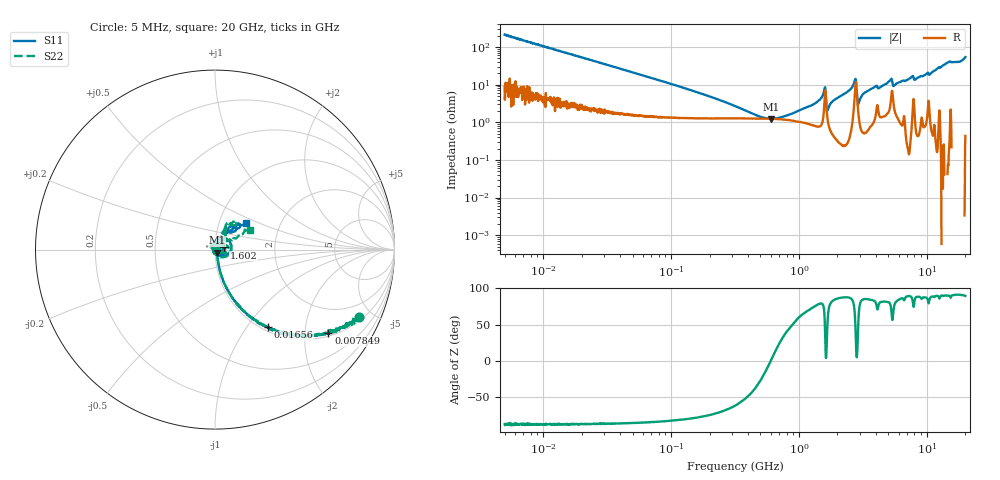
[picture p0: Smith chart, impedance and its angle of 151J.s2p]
!Keysight Technologies,P5008B,MY61100088,A.16.20.02
!Date: Wednesday, November 08, 2023 15:34:21
!Correction: S11(C  2-Port  )
!S21(C  2-Port  )
!S12(C  2-Port  )
!S22(C  2-Port  )
!S2P File: Measurements: S11, S21, S12, S22:Log Frequency Sweep
# Hz S  dB  R 50
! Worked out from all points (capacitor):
!   1601 points, 5 MHz to 20 GHz, reference 50 ohm
!   read as one part in series: C = 153 pF near 5.212 MHz
!   lowest |Z| = 1.23 ohm at 604.5 MHz (marker M1)
!   series resonance near 602.5 MHz, so ESL is about 460 pH
!   S11 on the Smith chart (normalised r, x): 5 MHz: 1.17, -4.19; 7.849 MHz: 1.09, -2.64; 16.56 MHz: 1.06, -1.27; 1.602 GHz: 1.11, +0.03; 20 GHz: 1.35, +0.42
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5000000  -1.03 -25.1  -7.45 62.5  -7.45 62.6  -1.03 -25.0
7849320  -2.11 -36.4  -4.54 51.6  -4.54 51.6  -2.11 -36.4
1.655836e7  -5.60 -55.5  -1.67 31.6  -1.66 31.6  -5.60 -55.6
1.995555e7  -6.76 -60.2  -1.23 27.3  -1.22 27.3  -6.76 -60.2
7.964482e7  -17.66 -76.7  -0.19 7.3  -0.19 7.3  -17.79 -77.0
3.162278e8  -29.20 -67.3  -0.12 1.1  -0.12 1.1  -31.44 -64.0
6.045204e8  -33.94 -58.0  -0.12 -0.6  -0.12 -0.6  -39.88 -13.4
1.2621e9  -44.82 -86.5  -0.14 -2.8  -0.14 -2.8  -35.82 80.8
1.399973e9  -52.34 173.2  -0.14 -3.3  -0.14 -3.3  -33.54 83.3
1.601965e9  -25.33 12.8  -0.67 -4.3  -0.67 -4.3  -24.26 20.9
1.722547e9  -38.19 -118.1  -0.16 -3.1  -0.16 -3.1  -43.61 107.4
2.760821e9  -20.64 32.2  -0.92 -8.4  -0.92 -8.4  -20.96 26.5
3.015158e9  -43.12 -161.9  -0.17 -5.2  -0.18 -5.2  -37.52 -109.6
3.361918e9  -36.72 103.7  -0.14 -6.9  -0.14 -6.9  -46.99 162.5
5.037181e9  -30.50 60.8  -0.16 -11.8  -0.16 -11.8  -27.52 32.2
6.070632e9  -42.06 -3.9  -0.15 -13.0  -0.15 -13.0  -45.95 58.5
7.165971e9  -38.79 25.2  -0.12 -15.6  -0.13 -15.6  -30.29 144.2
7.74541e9  -27.75 23.5  -0.28 -17.9  -0.28 -18.0  -32.63 87.4
8.591523e9  -41.64 -78.8  -0.07 -18.6  -0.07 -18.6  -40.28 -121.7
1.096177e10  -34.18 -9.0  -0.03 -24.5  -0.03 -24.6  -41.89 101.5
1.420512e10  -15.37 48.4  -0.05 -34.0  -0.05 -34.0  -15.55 59.6
2e10  -12.82 40.4  -0.33 -54.8  -0.33 -54.8  -13.06 29.0
